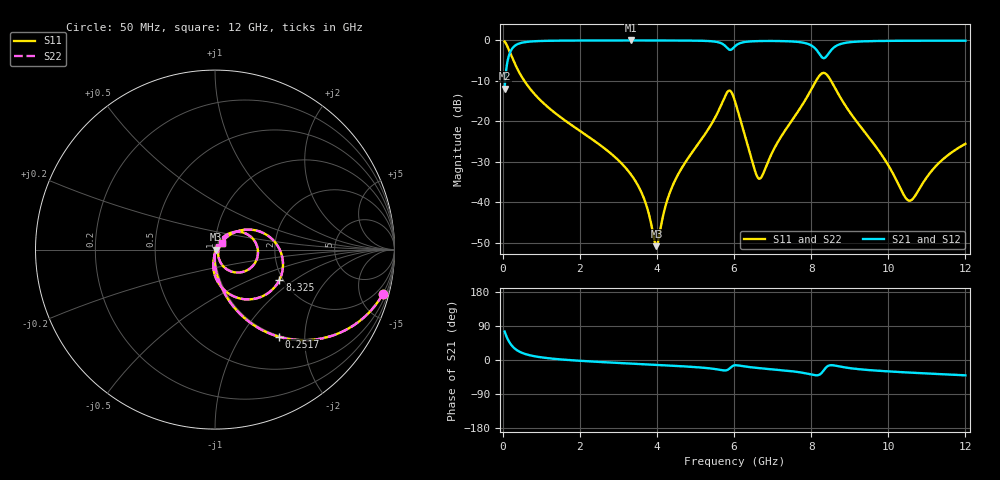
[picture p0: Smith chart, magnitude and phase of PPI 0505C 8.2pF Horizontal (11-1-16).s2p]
# MHz S MA R 50
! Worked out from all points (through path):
!   1601 points, 50 MHz to 12 GHz, reference 50 ohm
!   highest |S21| = -0.02 dB at 3.329 GHz (marker M1); lowest = -11.9 dB at 50 MHz (marker M2)
!   group delay of S21, straight-line fit = 12.2 ps
!   lowest |S11| = -50.8 dB at 3.986 GHz (marker M3), VSWR 1.01, Z = 50.3 - j0.0735 ohm
!   |S11| at or under -10 dB: 561.9 MHz to 8.126 GHz (7.564 GHz wide, 174 % of centre); 8.517 GHz to end of sweep
!   |S22| runs from -50.8 to -0.3 dB; largest |S21 - S12| = 0
!   S11 on the Smith chart (normalised r, x): 50 MHz: 0.98, -7.52; 251.7 MHz: 0.98, -1.49; 8.325 GHz: 1.92, -0.77; 12 GHz: 1.08, +0.08
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50  0.9671 -14.9  0.2543 75.1  0.2543 75.1  0.9671 -14.9
251.6562  0.6015 -53.8  0.7983 36.2  0.7983 36.2  0.6015 -53.8
677.375  0.2649 -76.6  0.9633 13.2  0.9633 13.2  0.2649 -76.6
2044.156  0.07414 -91.1  0.9955 -2.4  0.9955 -2.4  0.07414 -91.1
3328.781  0.02209 -93.6  0.9973 -9.5  0.9973 -9.5  0.02209 -93.6
3672.344  0.01096 -87.8  0.9972 -11.2  0.9972 -11.2  0.01096 -87.8
3986.031  0.002891 -14.6  0.9969 -12.8  0.9969 -12.8  0.002891 -14.6
4038.312  0.003435 17.3  0.9968 -13.1  0.9968 -13.1  0.003435 17.3
4269.844  0.01076 57.4  0.9963 -14.3  0.9963 -14.3  0.01076 57.4
4576.062  0.02339 63.5  0.9952 -16.0  0.9952 -16.0  0.02339 63.5
5442.438  0.09775 53.7  0.9726 -22.9  0.9726 -22.9  0.09775 53.7
5823.344  0.2292 9.9  0.8058 -26.5  0.8058 -26.5  0.2292 9.9
6025  0.1772 -46.2  0.8454 -13.9  0.8454 -13.9  0.1772 -46.2
6667.312  0.01966 -7.6  0.9805 -21.6  0.9805 -21.6  0.01966 -7.6
8019.156  0.256 24.3  0.8571 -38.7  0.8571 -38.7  0.256 24.3
8325.375  0.3967 -25.1  0.603 -27.3  0.603 -27.3  0.3967 -25.1
8489.688  0.3325 -56.6  0.7293 -13.9  0.7293 -13.9  0.3325 -56.6
8788.438  0.1865 -84.2  0.9095 -18.0  0.9095 -18.0  0.1865 -84.2
10013.31  0.0281 -91.7  0.9857 -30.1  0.9857 -30.1  0.0281 -91.7
10573.47  0.01055 -23.6  0.9889 -33.3  0.9889 -33.3  0.01055 -23.6
11268.06  0.02923 35.6  0.9901 -36.9  0.9901 -36.9  0.02923 35.6
12000  0.05291 40.9  0.9899 -40.4  0.9899 -40.4  0.05291 40.9
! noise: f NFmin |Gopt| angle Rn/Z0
50  0.0004341  0.8843  1.913  0.0008138
1372  0.004344  0.6971  4.924  0.002796
2701  0.007313  0.6552  8.965  0.004018
4031  0.01103  0.6594  12.99  0.006109
5360  0.0301  0.8191  17.12  0.03408
6682  0.03531  0.81  21.36  0.03741
8012  0.09998  0.9156  25.42  0.2486
9341  0.04735  0.8059  29.64  0.04744
1.067e+04  0.03243  0.6987  33.5  0.01935
1.2e+04  0.03064  0.6546  37.17  0.01526
